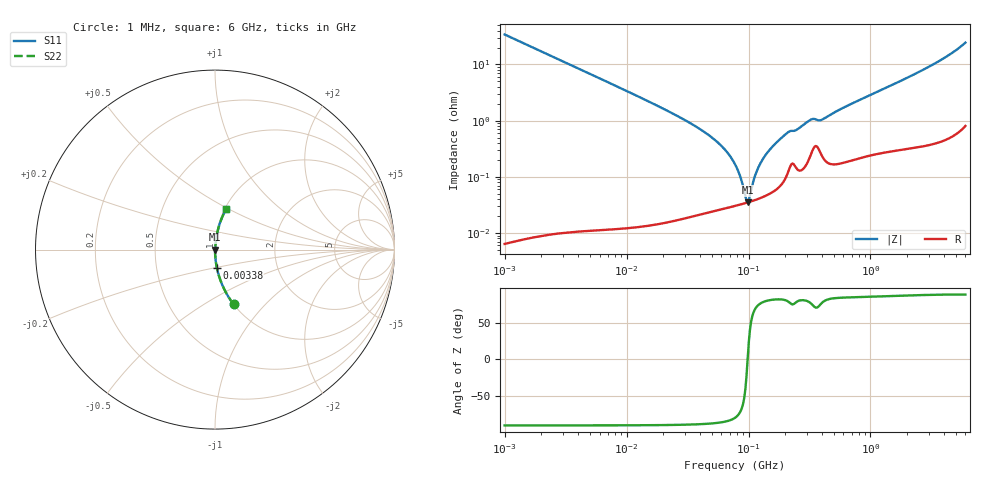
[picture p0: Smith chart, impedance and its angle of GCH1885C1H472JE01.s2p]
!Murata Part Number: GCH1885C1H472JE01
!These Parameters are Measured in Series Mode Connection
!Data Generated on Jun 19, 2026
!  o--ll--o
!Port1  Port2
!  o------o
!Operation Temp=25[degC], DC Bias Voltage=0[V]
!Freq. Start=1000[kHz] Stop=6[GHz] 401[Steps]
# Hz S RI R 50
!Freq.(Hz) S11(Real) S11(Imag) S21(Real) S21(Imag) S12(Real) S12(Imag) S22(Real) S22(Imag)
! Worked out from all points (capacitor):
!   401 points, 1 MHz to 6 GHz, reference 50 ohm
!   read as one part in series: C = 4.66 nF near 1.044 MHz
!   lowest |Z| = 35 mohm at 98.4 MHz (marker M1)
!   series resonance near 98.28 MHz, so ESL is about 560 pH
!   S11 on the Smith chart (normalised r, x): 1 MHz: 1.00, -0.68; 3.38 MHz: 1.00, -0.20; 6 GHz: 1.02, +0.49
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1000000  0.1043 -0.3056  0.8957 0.3056  0.8957 0.3056  0.1043 -0.3056
3380190  0.0102 -0.0998  0.9898 0.0998  0.9898 0.0998  0.0102 -0.0998
4293785  0.00635 -0.0788  0.9936 0.0788  0.9936 0.0788  0.00635 -0.0788
1.843659e7  0.000461 -0.0178  0.9995 0.0178  0.9995 0.0178  0.000461 -0.0178
3.316698e7  0.000274 -0.00905  0.9997 0.00905  0.9997 0.00905  0.000274 -0.00905
4.905945e7  0.000264 -0.00517  0.9997 0.00517  0.9997 0.00517  0.000264 -0.00517
6.368941e7  0.000282 -0.00307  0.9997 0.00307  0.9997 0.00307  0.000282 -0.00307
7.745967e7  0.000306 -0.00165  0.9997 0.00165  0.9997 0.00165  0.000306 -0.00165
8.450008e7  0.00032 -0.00104  0.9997 0.00104  0.9997 0.00104  0.00032 -0.00104
9.420718e7  0.00034 -0.000291  0.9997 0.000291  0.9997 0.000291  0.00034 -0.000291
9.83954e7  0.00035 8e-06  0.9997 -8e-06  0.9997 -8e-06  0.00035 8e-06
1.027698e8  0.00036 0.000307  0.9996 -0.000307  0.9996 -0.000307  0.00036 0.000307
1.121107e8  0.000384 0.00091  0.9996 -0.00091  0.9996 -0.00091  0.000384 0.00091
1.196694e8  0.000405 0.00137  0.9996 -0.00137  0.9996 -0.00137  0.000405 0.00137
1.455431e8  0.000493 0.0028  0.9995 -0.0028  0.9995 -0.0028  0.000493 0.0028
2.061188e8  0.0011 0.00586  0.9989 -0.00586  0.9989 -0.00586  0.0011 0.00586
2.506837e8  0.00141 0.00681  0.9986 -0.00681  0.9986 -0.00681  0.00141 0.00681
3.325952e8  0.00294 0.0102  0.9971 -0.0102  0.9971 -0.0102  0.00294 0.0102
4.045054e8  0.00236 0.0102  0.9976 -0.0102  0.9976 -0.0102  0.00236 0.0102
1.428092e9  0.00443 0.0405  0.9956 -0.0405  0.9956 -0.0405  0.00443 0.0405
3.483508e9  0.0154 0.1061  0.9846 -0.1061  0.9846 -0.1061  0.0154 0.1061
6e9  0.0628 0.2267  0.9372 -0.2267  0.9372 -0.2267  0.0628 0.2267
